| IBIS file generated by GenIBIS.pl Version 3.28
|   awr12csi3v3_fcbga161
[IBIS ver]   4.1
[File name]   awr12csi3v3_fcbga161.ibs
[File Rev]   1.1
[Date]   Wed Jan 25, 2017, 10:25:45
[Source]   Data created at Texas Instruments
[Notes]   1) NOT YET CHECKED BY IBISCK4. Once checked update notes
   section with any relevant information.
   2) Model not valid until this section updated.
   Some pins may contain selectors which are not valid options
   for that particular pin.
   Please refer to the device datasheet for information on picking
   the correct selector model, which depends on various software
   register configurations.
   Some pins are modeled as IO or tri-state for output mode.
   3) converted rev1.0 to rev1.1 by hand, part# change
[Disclaimer] Please be aware that in the absence of a written agreement,
   Texas Instruments (TI) assumes no liability for: 1) the
   accuracy of the IBIS models provided to your company, 2) the
   proper functioning of these IBIS models in your design or for
   any resulting applications, or, 3) infringement of patents,
   copyrights, or intellectual property rights resulting from
   your use of these IBIS models. TI provides IBIS models as a
   service to our customers and therefore reserves the right to
   limit distribution of the IBIS models.
[Copyright]   Property of Texas Instruments Incorporated. Unauthorised
   reproduction and/or distribution is strictly prohibited. This
   product is protected under copyright law and trade secret law
   as an unpublished work. Created 2010,(C) Copyright 2010,
   Texas Instruments Incorporated., All Rights Reserved. These
   commodities are under the U.S. Government distribution license
   control.As such,they are not to be re-exported without the
   prior approval of the U.S. Department of Commerce.
|   Component awr12csi3v3_fcbga161
[Component]   awr12csi3v3_fcbga161
[Manufacturer]   Texas Instruments.
| Source IO level model revisions
|Model   Revision   Date
|BC1833DV40DCPBFBP18LL_OD_FS_SSDLV  1.0   May 27, 2010
|DSIPHY_ADDON   0.8   July 13, 2011
|BC1833DV40DCPBFBP18LL_SSDLV   1.0   May 27, 2010
|BC1833DV40DCPBFBP18LL_SSDLH   1.0   May 27, 2010
|DSIPHY_CORE   0.8   July 13, 2011
[Package Model] awr12csi3v3_fcbga161
[Package]
|   typ   min   max
R_pkg   0.0921606365853659  25.6151E-3   196.84E-3
L_pkg   1.31603212195122E-009 0.489419E-9   2.33485E-9
C_pkg   4.95314675636342E-013 -0.0450383E-12   1.513E-12
[Pin]   signal_name   model_name
P1   ANALOGTEST1   NC
P2   ANALOGTEST2   NC
P3   ANALOGTEST3   NC
R2   ANALOGTEST4   NC
C13   ANAMUX   NC
F14   CLKM   NC
E14   CLKP   NC
G15   CSI2_TXP[0]   Model_78
J14   CSI2_CLKM   Model_25
L14   CSI2_TXM[3]   Model_78
H15   CSI2_TXP[1]   Model_25
K15   CSI2_TXP[2]   Model_78
J15   CSI2_CLKP   Model_25
L15   CSI2_TXP[3]   Model_78
G14   CSI2_TXM[0]   Model_78
H14   CSI2_TXM[1]   Model_25
K14   CSI2_TXM[2]   Model_78
B1   FM_CW_SYNCIN1   NC
D15   FM_CW_SYNCIN2   NC
B15   FM_CW_CLKOUT   NC
D1   FM_CW_SYNCOUT   NC
N4   GPIO_0   Selector_3
N7   GPIO_1   Selector_3
N13   GPIO_2   Selector_9
M14   HS_DEBUG1_M   NC
N15   HS_DEBUG2_P   NC
M15   HS_DEBUG1_P   NC
N14   HS_DEBUG2_M   NC
N9   MCU_CLKOUT   Selector_7
P4   MISO_2   Selector_7
P5   MISO_1   Selector_7
R3   MOSI_2   Selector_2
R8   MOSI_1   Selector_2
P7   NERROR_IN   Selector_1
N8   NERROR_OUT   Selector_6
P12   NRESET   NC
A14   OSC_CLKOUT   NC
P13   PMIC_CLKOUT   Selector_5
R12   QSPI[2]   Selector_4
P9   QSPI[1]   Selector_2
P10   QSPI[3]   Selector_2
R11   QSPI[0]   Selector_4
P8   QSPI_CS   Selector_7
R10   QSPI_CLK   Selector_7
G13   RESERVED   NC
N6   RS232_TX   Selector_7
N5   RS232_RX   Selector_2
M2   RX1   NC
K2   RX2   NC
H2   RX3   NC
F2   RX4   NC
R5   SPI_CLK_2   Selector_2
P6   SPI_HOST_INTR1   Selector_7
R4   SPI_CS_2   Selector_2
R7   SPI_CS_1   Selector_2
R9   SPI_CLK_1   Selector_2
N10   SYNC_IN   Selector_4
P11   SYNC_OUT   Selector_5
M13   TCK   Selector_4
H13   TDI   Selector_4
J13   TDO   Selector_5
L13   TMS   Selector_4
B4   TX1   NC
B6   TX2   NC
B8   TX3   NC
B10   VBGAP   NC
F13   VDDIN   NC
N11   VDDIN   NC
P15   VDDIN   NC
R6   VDDIN   NC
C2   VIN_13RF2   NC
D2   VIN_13RF2   NC
B12   VIN_18VCO   NC
G5   VIN_13RF1   NC
H5   VIN_13RF1   NC
J5   VIN_13RF1   NC
F5   VIN_18BB   NC
K5   VIN_18BB   NC
B11   VIN_18CLK   NC
R14   VIN_SRAM   NC
K13   VIOIN_18   NC
R13   VIOIN   NC
D13   VIOIN_18DIFF   NC
P14   VNWA   NC
A10   VOUT_14APLL1   NC
A2   VOUT_PA   NC
B2   VOUT_PA   NC
A13   VOUT_14SYNTH   NC
C14   VSENSE   NC
E10   VSS   NC
E11   VSS   NC
E5   VSS   NC
E6   VSS   NC
E8   VSS   NC
F11   VSS   NC
F9   VSS   NC
G10   VSS   NC
G6   VSS   NC
G7   VSS   NC
G8   VSS   NC
H11   VSS   NC
H7   VSS   NC
H9   VSS   NC
J10   VSS   NC
J6   VSS   NC
J7   VSS   NC
J8   VSS   NC
K10   VSS   NC
K11   VSS   NC
K7   VSS   NC
K8   VSS   NC
K9   VSS   NC
L10   VSS   NC
L5   VSS   NC
L6   VSS   NC
L8   VSS   NC
R15   VSS   NC
A15   VSSA   NC
A3   VSSA   NC
A5   VSSA   NC
A7   VSSA   NC
A9   VSSA   NC
B13   VSSA   NC
B14   VSSA   NC
B3   VSSA   NC
B5   VSSA   NC
B7   VSSA   NC
B9   VSSA   NC
C1   VSSA   NC
C15   VSSA   NC
C3   VSSA   NC
C4   VSSA   NC
C5   VSSA   NC
C6   VSSA   NC
C7   VSSA   NC
C8   VSSA   NC
C9   VSSA   NC
E1   VSSA   NC
E13   VSSA   NC
E15   VSSA   NC
E2   VSSA   NC
E3   VSSA   NC
F3   VSSA   NC
G1   VSSA   NC
G2   VSSA   NC
G3   VSSA   NC
H3   VSSA   NC
J1   VSSA   NC
J2   VSSA   NC
J3   VSSA   NC
K3   VSSA   NC
L1   VSSA   NC
L2   VSSA   NC
L3   VSSA   NC
M3   VSSA   NC
N1   VSSA   NC
N2   VSSA   NC
N3   VSSA   NC
R1   VSSA   NC
 A1   VSSA   NC
N12   WARM_RESET   Selector_8
[Diff Pin] inv_pin  vdiff  tdelay_typ
|Differential signal data for cell DSIPHY_ADDON
|CSI2_TXP[0]   CSI2_TXM[0]
G15   G14   200m   NA
|CSI2_TXP[2]   CSI2_TXM[2]
K15   K14   200m   NA
|CSI2_TXP[3]   CSI2_TXM[3]
L15   L14   200m   NA
|Differential signal data for cell DSIPHY_CORE
|CSI2_CLKP   CSI2_CLKM
J15   J14   200m   NA
|CSI2_TXP[1]   CSI2_TXM[1]
H15   H14   200m   NA
|   Usage INPUT#3.3#X#X#BC1833DV40DCPBFBP18LL_OD_FS_SSDLV.PAD
|   Base model BC1833DV40DCPBFBP18LL_OD_FS_SSDLV
[Model Selector] Selector_1
Model_10 I/O_OPEN_DRAIN,3.3V,WEAK_PU_ON,FAST,IND,5%,BC40D_V_PU_ON_5P_!SC1_3P3
Model_11 I/O_OPEN_DRAIN,3.3V,WEAK_PUPDOFF,FAST,IND,5%,BC40D_V_PUPDOFF_5P_!SC1_3
Model_12 I/O_OPEN_DRAIN,3.3V,WEAK_PU_ON,SLOW,IND,5%,BC40D_V_PU_ON_5P_SC1_3P3
Model_19 I/O_OPEN_DRAIN,3.3V,WEAK_PUPDOFF,SLOW,IND,10%,BC40D_V_PUPDOFF_10P_SC1_
Model_20 I/O_OPEN_DRAIN,3.3V,WEAK_PD_ON,FAST,IND,10%,BC40D_V_PD_ON_10P_!SC1_3P3
Model_21 I/O_OPEN_DRAIN,3.3V,WEAK_PD_ON,SLOW,IND,10%,BC40D_V_PD_ON_10P_SC1_3P3
Model_22 I/O_OPEN_DRAIN,3.3V,WEAK_PU_ON,FAST,IND,10%,BC40D_V_PU_ON_10P_!SC1_3P3
Model_23 I/O_OPEN_DRAIN,3.3V,WEAK_PUPDOFF,FAST,IND,10%,BC40D_V_PUPDOFF_10P_!SC1
Model_24 I/O_OPEN_DRAIN,3.3V,WEAK_PU_ON,SLOW,IND,10%,BC40D_V_PU_ON_10P_SC1_3P3
Model_7 I/O_OPEN_DRAIN,3.3V,WEAK_PUPDOFF,SLOW,IND,5%,BC40D_V_PUPDOFF_5P_SC1_3P
Model_8 I/O_OPEN_DRAIN,3.3V,WEAK_PD_ON,FAST,IND,5%,BC40D_V_PD_ON_5P_!SC1_3P3
Model_9 I/O_OPEN_DRAIN,3.3V,WEAK_PD_ON,SLOW,IND,5%,BC40D_V_PD_ON_5P_SC1_3P3
|   Usage INPUT#3.3#X#X#BC1833DV40DCPBFBP18LL_SSDLV.PAD
|   Base model BC1833DV40DCPBFBP18LL_SSDLV
[Model Selector] Selector_2
Model_60 I/O,3.3V,WEAK_PUPDOFF,SLOW,IND,5%,BC40D_V_PUPDOFF_5P_SC1_3P3
Model_61 I/O,3.3V,WEAK_PD_ON,FAST,IND,5%,BC40D_V_PD_ON_5P_!SC1_3P3
Model_62 I/O,3.3V,WEAK_PD_ON,SLOW,IND,5%,BC40D_V_PD_ON_5P_SC1_3P3
Model_63 I/O,3.3V,WEAK_PU_ON,FAST,IND,5%,BC40D_V_PU_ON_5P_!SC1_3P3
Model_64 I/O,3.3V,WEAK_PUPDOFF,FAST,IND,5%,BC40D_V_PUPDOFF_5P_!SC1_3P3
Model_65 I/O,3.3V,WEAK_PU_ON,SLOW,IND,5%,BC40D_V_PU_ON_5P_SC1_3P3
Model_72 I/O,3.3V,WEAK_PUPDOFF,SLOW,IND,10%,BC40D_V_PUPDOFF_10P_SC1_3P3
Model_73 I/O,3.3V,WEAK_PD_ON,FAST,IND,10%,BC40D_V_PD_ON_10P_!SC1_3P3
Model_74 I/O,3.3V,WEAK_PD_ON,SLOW,IND,10%,BC40D_V_PD_ON_10P_SC1_3P3
Model_75 I/O,3.3V,WEAK_PU_ON,FAST,IND,10%,BC40D_V_PU_ON_10P_!SC1_3P3
Model_76 I/O,3.3V,WEAK_PUPDOFF,FAST,IND,10%,BC40D_V_PUPDOFF_10P_!SC1_3P3
Model_77 I/O,3.3V,WEAK_PU_ON,SLOW,IND,10%,BC40D_V_PU_ON_10P_SC1_3P3
|   Usage I/O#3.3#X#X#BC1833DV40DCPBFBP18LL_SSDLV.PAD
|   Base model BC1833DV40DCPBFBP18LL_SSDLV
[Model Selector] Selector_3
Model_60 I/O,3.3V,WEAK_PUPDOFF,SLOW,IND,5%,BC40D_V_PUPDOFF_5P_SC1_3P3
Model_61 I/O,3.3V,WEAK_PD_ON,FAST,IND,5%,BC40D_V_PD_ON_5P_!SC1_3P3
Model_62 I/O,3.3V,WEAK_PD_ON,SLOW,IND,5%,BC40D_V_PD_ON_5P_SC1_3P3
Model_63 I/O,3.3V,WEAK_PU_ON,FAST,IND,5%,BC40D_V_PU_ON_5P_!SC1_3P3
Model_64 I/O,3.3V,WEAK_PUPDOFF,FAST,IND,5%,BC40D_V_PUPDOFF_5P_!SC1_3P3
Model_65 I/O,3.3V,WEAK_PU_ON,SLOW,IND,5%,BC40D_V_PU_ON_5P_SC1_3P3
Model_72 I/O,3.3V,WEAK_PUPDOFF,SLOW,IND,10%,BC40D_V_PUPDOFF_10P_SC1_3P3
Model_73 I/O,3.3V,WEAK_PD_ON,FAST,IND,10%,BC40D_V_PD_ON_10P_!SC1_3P3
Model_74 I/O,3.3V,WEAK_PD_ON,SLOW,IND,10%,BC40D_V_PD_ON_10P_SC1_3P3
Model_75 I/O,3.3V,WEAK_PU_ON,FAST,IND,10%,BC40D_V_PU_ON_10P_!SC1_3P3
Model_76 I/O,3.3V,WEAK_PUPDOFF,FAST,IND,10%,BC40D_V_PUPDOFF_10P_!SC1_3P3
Model_77 I/O,3.3V,WEAK_PU_ON,SLOW,IND,10%,BC40D_V_PU_ON_10P_SC1_3P3
|   Usage INPUT#3.3#X#X#BC1833DV40DCPBFBP18LL_SSDLH.PAD
|   Base model BC1833DV40DCPBFBP18LL_SSDLH
[Model Selector] Selector_4
Model_36 I/O,3.3V,WEAK_PUPDOFF,SLOW,IND,5%,BC40D_H_PUPDOFF_5P_SC1_3P3
Model_37 I/O,3.3V,WEAK_PD_ON,FAST,IND,5%,BC40D_H_PD_ON_5P_!SC1_3P3
Model_38 I/O,3.3V,WEAK_PD_ON,SLOW,IND,5%,BC40D_H_PD_ON_5P_SC1_3P3
Model_39 I/O,3.3V,WEAK_PU_ON,FAST,IND,5%,BC40D_H_PU_ON_5P_!SC1_3P3
Model_40 I/O,3.3V,WEAK_PUPDOFF,FAST,IND,5%,BC40D_H_PUPDOFF_5P_!SC1_3P3
Model_41 I/O,3.3V,WEAK_PU_ON,SLOW,IND,5%,BC40D_H_PU_ON_5P_SC1_3P3
Model_48 I/O,3.3V,WEAK_PUPDOFF,SLOW,IND,10%,BC40D_H_PUPDOFF_10P_SC1_3P3
Model_49 I/O,3.3V,WEAK_PD_ON,FAST,IND,10%,BC40D_H_PD_ON_10P_!SC1_3P3
Model_50 I/O,3.3V,WEAK_PD_ON,SLOW,IND,10%,BC40D_H_PD_ON_10P_SC1_3P3
Model_51 I/O,3.3V,WEAK_PU_ON,FAST,IND,10%,BC40D_H_PU_ON_10P_!SC1_3P3
Model_52 I/O,3.3V,WEAK_PUPDOFF,FAST,IND,10%,BC40D_H_PUPDOFF_10P_!SC1_3P3
Model_53 I/O,3.3V,WEAK_PU_ON,SLOW,IND,10%,BC40D_H_PU_ON_10P_SC1_3P3
|   Usage OUTPUT#3.3#X#X#BC1833DV40DCPBFBP18LL_SSDLH.PAD
|   Base model BC1833DV40DCPBFBP18LL_SSDLH
[Model Selector] Selector_5
Model_36 I/O,3.3V,WEAK_PUPDOFF,SLOW,IND,5%,BC40D_H_PUPDOFF_5P_SC1_3P3
Model_37 I/O,3.3V,WEAK_PD_ON,FAST,IND,5%,BC40D_H_PD_ON_5P_!SC1_3P3
Model_38 I/O,3.3V,WEAK_PD_ON,SLOW,IND,5%,BC40D_H_PD_ON_5P_SC1_3P3
Model_39 I/O,3.3V,WEAK_PU_ON,FAST,IND,5%,BC40D_H_PU_ON_5P_!SC1_3P3
Model_40 I/O,3.3V,WEAK_PUPDOFF,FAST,IND,5%,BC40D_H_PUPDOFF_5P_!SC1_3P3
Model_41 I/O,3.3V,WEAK_PU_ON,SLOW,IND,5%,BC40D_H_PU_ON_5P_SC1_3P3
Model_48 I/O,3.3V,WEAK_PUPDOFF,SLOW,IND,10%,BC40D_H_PUPDOFF_10P_SC1_3P3
Model_49 I/O,3.3V,WEAK_PD_ON,FAST,IND,10%,BC40D_H_PD_ON_10P_!SC1_3P3
Model_50 I/O,3.3V,WEAK_PD_ON,SLOW,IND,10%,BC40D_H_PD_ON_10P_SC1_3P3
Model_51 I/O,3.3V,WEAK_PU_ON,FAST,IND,10%,BC40D_H_PU_ON_10P_!SC1_3P3
Model_52 I/O,3.3V,WEAK_PUPDOFF,FAST,IND,10%,BC40D_H_PUPDOFF_10P_!SC1_3P3
Model_53 I/O,3.3V,WEAK_PU_ON,SLOW,IND,10%,BC40D_H_PU_ON_10P_SC1_3P3
|   Usage OUTPUT#3.3#X#X#BC1833DV40DCPBFBP18LL_OD_FS_SSDLV.PAD
|   Base model BC1833DV40DCPBFBP18LL_OD_FS_SSDLV
[Model Selector] Selector_6
Model_10 I/O_OPEN_DRAIN,3.3V,WEAK_PU_ON,FAST,IND,5%,BC40D_V_PU_ON_5P_!SC1_3P3
Model_11 I/O_OPEN_DRAIN,3.3V,WEAK_PUPDOFF,FAST,IND,5%,BC40D_V_PUPDOFF_5P_!SC1_3
Model_12 I/O_OPEN_DRAIN,3.3V,WEAK_PU_ON,SLOW,IND,5%,BC40D_V_PU_ON_5P_SC1_3P3
Model_19 I/O_OPEN_DRAIN,3.3V,WEAK_PUPDOFF,SLOW,IND,10%,BC40D_V_PUPDOFF_10P_SC1_
Model_20 I/O_OPEN_DRAIN,3.3V,WEAK_PD_ON,FAST,IND,10%,BC40D_V_PD_ON_10P_!SC1_3P3
Model_21 I/O_OPEN_DRAIN,3.3V,WEAK_PD_ON,SLOW,IND,10%,BC40D_V_PD_ON_10P_SC1_3P3
Model_22 I/O_OPEN_DRAIN,3.3V,WEAK_PU_ON,FAST,IND,10%,BC40D_V_PU_ON_10P_!SC1_3P3
Model_23 I/O_OPEN_DRAIN,3.3V,WEAK_PUPDOFF,FAST,IND,10%,BC40D_V_PUPDOFF_10P_!SC1
Model_24 I/O_OPEN_DRAIN,3.3V,WEAK_PU_ON,SLOW,IND,10%,BC40D_V_PU_ON_10P_SC1_3P3
Model_7 I/O_OPEN_DRAIN,3.3V,WEAK_PUPDOFF,SLOW,IND,5%,BC40D_V_PUPDOFF_5P_SC1_3P
Model_8 I/O_OPEN_DRAIN,3.3V,WEAK_PD_ON,FAST,IND,5%,BC40D_V_PD_ON_5P_!SC1_3P3
Model_9 I/O_OPEN_DRAIN,3.3V,WEAK_PD_ON,SLOW,IND,5%,BC40D_V_PD_ON_5P_SC1_3P3
|   Usage OUTPUT#3.3#X#X#BC1833DV40DCPBFBP18LL_SSDLV.PAD
|   Base model BC1833DV40DCPBFBP18LL_SSDLV
[Model Selector] Selector_7
Model_60 I/O,3.3V,WEAK_PUPDOFF,SLOW,IND,5%,BC40D_V_PUPDOFF_5P_SC1_3P3
Model_61 I/O,3.3V,WEAK_PD_ON,FAST,IND,5%,BC40D_V_PD_ON_5P_!SC1_3P3
Model_62 I/O,3.3V,WEAK_PD_ON,SLOW,IND,5%,BC40D_V_PD_ON_5P_SC1_3P3
Model_63 I/O,3.3V,WEAK_PU_ON,FAST,IND,5%,BC40D_V_PU_ON_5P_!SC1_3P3
Model_64 I/O,3.3V,WEAK_PUPDOFF,FAST,IND,5%,BC40D_V_PUPDOFF_5P_!SC1_3P3
Model_65 I/O,3.3V,WEAK_PU_ON,SLOW,IND,5%,BC40D_V_PU_ON_5P_SC1_3P3
Model_72 I/O,3.3V,WEAK_PUPDOFF,SLOW,IND,10%,BC40D_V_PUPDOFF_10P_SC1_3P3
Model_73 I/O,3.3V,WEAK_PD_ON,FAST,IND,10%,BC40D_V_PD_ON_10P_!SC1_3P3
Model_74 I/O,3.3V,WEAK_PD_ON,SLOW,IND,10%,BC40D_V_PD_ON_10P_SC1_3P3
Model_75 I/O,3.3V,WEAK_PU_ON,FAST,IND,10%,BC40D_V_PU_ON_10P_!SC1_3P3
Model_76 I/O,3.3V,WEAK_PUPDOFF,FAST,IND,10%,BC40D_V_PUPDOFF_10P_!SC1_3P3
Model_77 I/O,3.3V,WEAK_PU_ON,SLOW,IND,10%,BC40D_V_PU_ON_10P_SC1_3P3
|   Usage I/O#3.3#X#X#BC1833DV40DCPBFBP18LL_OD_FS_SSDLV.PAD
|   Base model BC1833DV40DCPBFBP18LL_OD_FS_SSDLV
[Model Selector] Selector_8
Model_10 I/O_OPEN_DRAIN,3.3V,WEAK_PU_ON,FAST,IND,5%,BC40D_V_PU_ON_5P_!SC1_3P3
Model_11 I/O_OPEN_DRAIN,3.3V,WEAK_PUPDOFF,FAST,IND,5%,BC40D_V_PUPDOFF_5P_!SC1_3
Model_12 I/O_OPEN_DRAIN,3.3V,WEAK_PU_ON,SLOW,IND,5%,BC40D_V_PU_ON_5P_SC1_3P3
Model_19 I/O_OPEN_DRAIN,3.3V,WEAK_PUPDOFF,SLOW,IND,10%,BC40D_V_PUPDOFF_10P_SC1_
Model_20 I/O_OPEN_DRAIN,3.3V,WEAK_PD_ON,FAST,IND,10%,BC40D_V_PD_ON_10P_!SC1_3P3
Model_21 I/O_OPEN_DRAIN,3.3V,WEAK_PD_ON,SLOW,IND,10%,BC40D_V_PD_ON_10P_SC1_3P3
Model_22 I/O_OPEN_DRAIN,3.3V,WEAK_PU_ON,FAST,IND,10%,BC40D_V_PU_ON_10P_!SC1_3P3
Model_23 I/O_OPEN_DRAIN,3.3V,WEAK_PUPDOFF,FAST,IND,10%,BC40D_V_PUPDOFF_10P_!SC1
Model_24 I/O_OPEN_DRAIN,3.3V,WEAK_PU_ON,SLOW,IND,10%,BC40D_V_PU_ON_10P_SC1_3P3
Model_7 I/O_OPEN_DRAIN,3.3V,WEAK_PUPDOFF,SLOW,IND,5%,BC40D_V_PUPDOFF_5P_SC1_3P
Model_8 I/O_OPEN_DRAIN,3.3V,WEAK_PD_ON,FAST,IND,5%,BC40D_V_PD_ON_5P_!SC1_3P3
Model_9 I/O_OPEN_DRAIN,3.3V,WEAK_PD_ON,SLOW,IND,5%,BC40D_V_PD_ON_5P_SC1_3P3
|   Usage I/O#3.3#X#X#BC1833DV40DCPBFBP18LL_SSDLH.PAD
|   Base model BC1833DV40DCPBFBP18LL_SSDLH
[Model Selector] Selector_9
Model_36 I/O,3.3V,WEAK_PUPDOFF,SLOW,IND,5%,BC40D_H_PUPDOFF_5P_SC1_3P3
Model_37 I/O,3.3V,WEAK_PD_ON,FAST,IND,5%,BC40D_H_PD_ON_5P_!SC1_3P3
Model_38 I/O,3.3V,WEAK_PD_ON,SLOW,IND,5%,BC40D_H_PD_ON_5P_SC1_3P3
Model_39 I/O,3.3V,WEAK_PU_ON,FAST,IND,5%,BC40D_H_PU_ON_5P_!SC1_3P3
Model_40 I/O,3.3V,WEAK_PUPDOFF,FAST,IND,5%,BC40D_H_PUPDOFF_5P_!SC1_3P3
Model_41 I/O,3.3V,WEAK_PU_ON,SLOW,IND,5%,BC40D_H_PU_ON_5P_SC1_3P3
Model_48 I/O,3.3V,WEAK_PUPDOFF,SLOW,IND,10%,BC40D_H_PUPDOFF_10P_SC1_3P3
Model_49 I/O,3.3V,WEAK_PD_ON,FAST,IND,10%,BC40D_H_PD_ON_10P_!SC1_3P3
Model_50 I/O,3.3V,WEAK_PD_ON,SLOW,IND,10%,BC40D_H_PD_ON_10P_SC1_3P3
Model_51 I/O,3.3V,WEAK_PU_ON,FAST,IND,10%,BC40D_H_PU_ON_10P_!SC1_3P3
Model_52 I/O,3.3V,WEAK_PUPDOFF,FAST,IND,10%,BC40D_H_PUPDOFF_10P_!SC1_3P3
Model_53 I/O,3.3V,WEAK_PU_ON,SLOW,IND,10%,BC40D_H_PU_ON_10P_SC1_3P3
| Package model definition
[Define Package Model]  awr12csi3v3_fcbga161
[Manufacturer]   Texas Instruments.
[OEM]   Texas Instruments.
[Description]   awr12csi3v3_fcbga161 package model generated by GenIBIS.pl
[Number Of Pins]   41
[Pin Numbers]
G15   | 1 CSI2_TXP[0]   OUTPUT
J14   | 2 CSI2_CLKM   OUTPUT
L14   | 3 CSI2_TXM[3]   OUTPUT
H15   | 4 CSI2_TXP[1]   OUTPUT
K15   | 5 CSI2_TXP[2]   OUTPUT
J15   | 6 CSI2_CLKP   OUTPUT
L15   | 7 CSI2_TXP[3]   OUTPUT
G14   | 8 CSI2_TXM[0]   OUTPUT
H14   | 9 CSI2_TXM[1]   OUTPUT
K14   | 10 CSI2_TXM[2]   OUTPUT
N4   | 11 GPIO_0   I/O
N7   | 12 GPIO_1   I/O
N13   | 13 GPIO_2   I/O
N9   | 14 MCU_CLKOUT   OUTPUT
P4   | 15 MISO_2   OUTPUT
P5   | 16 MISO_1   OUTPUT
R3   | 17 MOSI_2   INPUT
R8   | 18 MOSI_1   INPUT
P7   | 19 NERROR_IN   INPUT
N8   | 20 NERROR_OUT   OUTPUT
P13   | 21 PMIC_CLKOUT   OUTPUT
R12   | 22 QSPI[2]   INPUT
P9   | 23 QSPI[1]   INPUT
P10   | 24 QSPI[3]   INPUT
R11   | 25 QSPI[0]   INPUT
P8   | 26 QSPI_CS   OUTPUT
R10   | 27 QSPI_CLK   OUTPUT
N6   | 28 RS232_TX   OUTPUT
N5   | 29 RS232_RX   INPUT
R5   | 30 SPI_CLK_2   INPUT
P6   | 31 SPI_HOST_INTR1   OUTPUT
R4   | 32 SPI_CS_2   INPUT
R7   | 33 SPI_CS_1   INPUT
R9   | 34 SPI_CLK_1   INPUT
N10   | 35 SYNC_IN   INPUT
P11   | 36 SYNC_OUT   OUTPUT
M13   | 37 TCK   INPUT
H13   | 38 TDI   INPUT
J13   | 39 TDO   OUTPUT
L13   | 40 TMS   INPUT
N12   | 41 WARM_RESET   I/O
[Model Data]
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[End Model Data]
[End Package Model]
| Models and submodels in the file (38): Model_7 (I/O_open_drain), Model_8 (I/O_open_drain), Model_9 (I/O_open_drain), Model_10 (I/O_open_drain), Model_11 (I/O_open_drain), Model_12 (I/O_open_drain), Model_19 (I/O_open_drain), Model_20 (I/O_open_drain), Model_21 (I/O_open_drain), Model_22 (I/O_open_drain), Model_23 (I/O_open_drain), Model_24 (I/O_open_drain), Model_25 (Output), Model_36 (I/O), Model_37 (I/O), Model_38 (I/O), Model_39 (I/O), Model_40 (I/O), Model_41 (I/O), Model_48 (I/O), Model_49 (I/O), Model_50 (I/O), Model_51 (I/O), Model_52 (I/O), Model_53 (I/O), Model_60 (I/O), Model_61 (I/O), Model_62 (I/O), Model_63 (I/O), Model_64 (I/O), Model_65 (I/O), Model_72 (I/O), Model_73 (I/O), Model_74 (I/O), Model_75 (I/O), Model_76 (I/O), Model_77 (I/O), Model_78 (Output)
